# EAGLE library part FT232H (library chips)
Single Channel USB to Multipurpose I/O IC
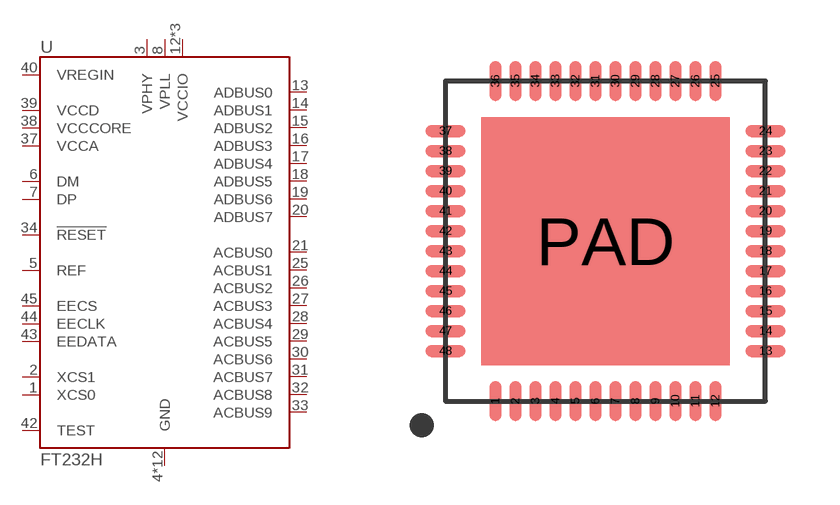
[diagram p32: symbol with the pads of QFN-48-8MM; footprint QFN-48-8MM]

Designator prefix U

## FT232HQ (DIGIKEY: 768-1102-1-ND; MOUSER: 895-FT232HQ-REEL; NEWARK: 65W8039)  [QFN-48-8MM]
1  XCS0
2  XCS1
3  VPHY
4  GND
5  REF
6  DM
7  DP
8  VPLL
9  GND
10  GND
11  GND
12  VCCIO
13  ADBUS0
14  ADBUS1
15  ADBUS2
16  ADBUS3
17  ADBUS4
18  ADBUS5
19  ADBUS6
20  ADBUS7
21  ACBUS0
22  GND
23  GND
24  VCCIO
25  ACBUS1
26  ACBUS2
27  ACBUS3
28  ACBUS4
29  ACBUS5
30  ACBUS6
31  ACBUS7
32  ACBUS8
33  ACBUS9
34  !RESET
35  GND
36  GND
37  VCCA
38  VCCCORE
39  VCCD
40  VREGIN
41  GND
42  TEST
43  EEDATA
44  EECLK
45  EECS
46  VCCIO
47  GND
48  GND
PAD  GND

## Footprint QFN-48-8MM (pad centres in mm)
smd 0.3 x 1: 1 -2.75,-4; 2 -2.25,-4; 3 -1.75,-4; 4 -1.25,-4; 5 -0.75,-4; 6 -0.25,-4; 7 0.25,-4; 8 0.75,-4; 9 1.25,-4; 10 1.75,-4; 11 2.25,-4; 12 2.75,-4; 25 2.75,4; 26 2.25,4; 27 1.75,4; 28 1.25,4; 29 0.75,4; 30 0.25,4; 31 -0.25,4; 32 -0.75,4; 33 -1.25,4; 34 -1.75,4; 35 -2.25,4; 36 -2.75,4
smd 1 x 0.3: 13 4,-2.75; 14 4,-2.25; 15 4,-1.75; 16 4,-1.25; 17 4,-0.75; 18 4,-0.25; 19 4,0.25; 20 4,0.75; 21 4,1.25; 22 4,1.75; 23 4,2.25; 24 4,2.75; 37 -4,2.75; 38 -4,2.25; 39 -4,1.75; 40 -4,1.25; 41 -4,0.75; 42 -4,0.25; 43 -4,-0.25; 44 -4,-0.75; 45 -4,-1.25; 46 -4,-1.75; 47 -4,-2.25; 48 -4,-2.75
smd 6.2 x 6.2: PAD 0,0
